|   IBIS model for TI xxx DSP
[IBIS Ver]   5.1
[Disclaimer]   Please be aware that in the absence of a written agreement
|   Texas Instruments(TI) assumes no liability for:
|   (1) The accuracy of the IBIS models provided to your company,
|   however, the IBIS model is compliant to industry standard
|   IQ Level 2a.  Refer to IBIS Quality Section below for
|   for full details.
|   (2) The proper functioning of these Models in your design
|   or for any resulting applications
|   (3) Infringement of patents, copyrights or intellectual
|   property rights resulting from your use of these
|   models.
|   TI provides IBIS Models as a service to our customers and
|   therefore reserves the right to limit distribution of the
|   Models.  The information is subject to change without notice.
[File Name]  am64_ani.ibs
[File Rev]   0.1
|   - Initial version
[Date]   3 Nov 2025
[Source]   Texas Instruments Incorporated
[Copyright]   Property of Texas Instruments Incorporated.
|   Unauthorized reproduction and/or distribution is strictly.
|   prohibited.
|   This product is protected under copyright law and trade
|   secret law as an unpublished work.
|   Created 2012,(C) Copyright 1999-2012,
|   Texas Instruments Incorporated., All Rights Reserved.
|   These commodities are under the U.S. Government
|   distribution license control. As such,they are not to be
|   re-exported without the prior approval of the U.S.
|   Department of Commerce.
[Notes]
   This file does not include AMI models for SerDes based links.
   For SerDes simulations use Texas Instruments IBIS AMI models
   Some IV curves contain Non monotonic data points.
|   Revision History
|   GERNERAL COMMENT: All IBIS Quality Notes below reflect latest release
|   and version of IBIS File
|   File passes ibischk5.1 and ibischk6 with 0 errors and 66 warnings
|   Component AM64
[Component] AM64
[Manufacturer] Texas Instruments
[Package]
|Variable   Typ   Min   Max
R_pkg   0.36429   0.078021   0.69181
L_pkg   2.771e-9   9.357e-10   5.062e-9
C_pkg   1.024e-12   5.807e-13   1.505e-12
[Package Model]   am64_ani_pkg
[Pin]  Signal_name   model_name
G20	ADC0_AIN0		NC
F20	ADC0_AIN1		NC
E21	ADC0_AIN2		NC
D20	ADC0_AIN3		NC
G21	ADC0_AIN4		NC
F21	ADC0_AIN5		NC
F19	ADC0_AIN6		NC
E20	ADC0_AIN7		NC
J16	ADC0_REFN		NC
J15	ADC0_REFP		NC
G13	ATEST0			NC
D2	DDR0_A0			DDR_SE
C5	DDR0_A1			DDR_SE
K3	DDR0_A10		DDR_SE
J1	DDR0_A11		DDR_SE
M5	DDR0_A12		DDR_SE
K4	DDR0_A13		DDR_SE
E2	DDR0_A2			DDR_SE
D4	DDR0_A3			DDR_SE
D3	DDR0_A4			DDR_SE
F2	DDR0_A5			DDR_SE
J2	DDR0_A6			DDR_SE
L5	DDR0_A7			DDR_SE
J3	DDR0_A8			DDR_SE
J4	DDR0_A9			DDR_SE
H2	DDR0_ACT_N		DDR_SE
H1	DDR0_ALERT_N   DDR_SE
K2	DDR0_ATB0		DDR_SE
K1	DDR0_ATB1		DDR_SE
G4	DDR0_BA0		DDR_SE
G5	DDR0_BA1		DDR_SE
G2	DDR0_BG0		DDR_SE
H3	DDR0_BG1		DDR_SE
H5	DDR0_CAL0		DDR_SE
J5	DDR0_CAS_N		DDR_SE
F1	DDR0_CK0		DDR_DIFF
E1	DDR0_CK0_N		DDR_DIFF
F4	DDR0_CKE0		DDR_SE
F3	DDR0_CKE1		DDR_SE
E3	DDR0_CS0_N		DDR_SE
E4	DDR0_CS1_N		DDR_SE
B2	DDR0_DM0		DDR_SE
M2	DDR0_DM1   DDR_SE
A3	DDR0_DQ0   DDR_SE
A2	DDR0_DQ1   DDR_SE
L2	DDR0_DQ10   DDR_SE
M3	DDR0_DQ11   DDR_SE
N4	DDR0_DQ12   DDR_SE
N3	DDR0_DQ13   DDR_SE
M4	DDR0_DQ14   DDR_SE
N2	DDR0_DQ15   DDR_SE
B5	DDR0_DQ2   DDR_SE
A4	DDR0_DQ3   DDR_SE
B3	DDR0_DQ4   DDR_SE
C4	DDR0_DQ5   DDR_SE
C2	DDR0_DQ6   DDR_SE
B4	DDR0_DQ7   DDR_SE
N5	DDR0_DQ8   DDR_SE
L4	DDR0_DQ9   DDR_SE
C1	DDR0_DQS0   DDR_DIFF
B1	DDR0_DQS0_N   DDR_DIFF
N1	DDR0_DQS1   DDR_DIFF
M1	DDR0_DQS1_N   DDR_DIFF
E5	DDR0_ODT0   DDR_SE
F5	DDR0_ODT1   DDR_SE
K5	DDR0_PAR   DDR_SE
F6	DDR0_RAS_N   DDR_SE
D5	DDR0_RESET0_N   DDR_SE
H4	DDR0_WE_N   DDR_SE
D18	ECAP0_IN_APWM_OUT	LVCMOS_V
D10	EMU0   LVCMOS_V
E10	EMU1   LVCMOS_V
A19	EXT_REFCLK1   LVCMOS_V
C19	EXTINTN   IIC_V
T20	GPMC0_AD0   LVCMOS_H
U21	GPMC0_AD1   LVCMOS_H
R16	GPMC0_AD10   LVCMOS_H
W20	GPMC0_AD11   LVCMOS_H
W21	GPMC0_AD12   LVCMOS_H
V18	GPMC0_AD13   LVCMOS_H
Y21	GPMC0_AD14   LVCMOS_H
Y20	GPMC0_AD15   LVCMOS_H
T18	GPMC0_AD2   LVCMOS_H
U20	GPMC0_AD3   LVCMOS_H
U18	GPMC0_AD4   LVCMOS_H
U19	GPMC0_AD5   LVCMOS_H
V20	GPMC0_AD6   LVCMOS_H
V21	GPMC0_AD7   LVCMOS_H
V19	GPMC0_AD8   LVCMOS_H
T17	GPMC0_AD9   LVCMOS_H
P16	GPMC0_ADVN_ALE   LVCMOS_H
P17	GPMC0_BE0N_CLE   LVCMOS_H
T19	GPMC0_BE1N   LVCMOS_H
R17	GPMC0_CLK   LVCMOS_H
R19	GPMC0_CSN0   LVCMOS_H
R20	GPMC0_CSN1   LVCMOS_H
P19	GPMC0_CSN2   LVCMOS_H
R21	GPMC0_CSN3   LVCMOS_H
N17	GPMC0_DIR   LVCMOS_H
R18	GPMC0_OEN_REN   LVCMOS_H
W19	GPMC0_WAIT0   LVCMOS_H
Y18	GPMC0_WAIT1   LVCMOS_H
T21	GPMC0_WEN   LVCMOS_H
N16	GPMC0_WPN   LVCMOS_H
A18	I2C0_SCL   IIC_V
B18	I2C0_SDA   IIC_V
C18	I2C1_SCL   LVCMOS_V
B19	I2C1_SDA   LVCMOS_V
H16	IFORCE   NC
B17	MCAN0_RX   LVCMOS_V
A17	MCAN0_TX   LVCMOS_V
D17	MCAN1_RX   LVCMOS_V
C17	MCAN1_TX   LVCMOS_V
E9	MCU_I2C0_SCL   IIC_V
A10	MCU_I2C0_SDA   IIC_V
A11	MCU_I2C1_SCL   LVCMOS_V
B10	MCU_I2C1_SDA   LVCMOS_V
C21	MCU_OSC0_XI   NC
B20	MCU_OSC0_XO   NC
B21	MCU_PORZ   RESET_H
B13	MCU_RESETSTATZ   LVCMOS_V
B12	MCU_RESETZ   LVCMOS_V
A20	MCU_SAFETY_ERRORN	LVCMOS_V
E6	MCU_SPI0_CLK   LVCMOS_V
D6	MCU_SPI0_CS0   LVCMOS_V
C6	MCU_SPI0_CS1   LVCMOS_V
E7	MCU_SPI0_D0   LVCMOS_V
B6	MCU_SPI0_D1   LVCMOS_V
D7	MCU_SPI1_CLK   LVCMOS_V
A7	MCU_SPI1_CS0   LVCMOS_V
B7	MCU_SPI1_CS1   LVCMOS_V
C7	MCU_SPI1_D0   LVCMOS_V
C8	MCU_SPI1_D1   LVCMOS_V
D8	MCU_UART0_CTSN   LVCMOS_V
E8	MCU_UART0_RTSN   LVCMOS_V
A9	MCU_UART0_RXD   LVCMOS_V
A8	MCU_UART0_TXD   LVCMOS_V
B8	MCU_UART1_CTSN   LVCMOS_V
B9	MCU_UART1_RTSN   LVCMOS_V
C9	MCU_UART1_RXD   LVCMOS_V
D9	MCU_UART1_TXD   LVCMOS_V
F18	MMC0_CALPAD   EMMC
G18	MMC0_CLK   EMMC
J21	MMC0_CMD   EMMC
K20	MMC0_DAT0   EMMC
J20	MMC0_DAT1   EMMC
J18	MMC0_DAT2   EMMC
J17	MMC0_DAT3   EMMC
H17	MMC0_DAT4   EMMC
H19	MMC0_DAT5   EMMC
H18	MMC0_DAT6   EMMC
G17	MMC0_DAT7   EMMC
G19	MMC0_DS   EMMC
F17	MMC0_VCTRL_TP   EMMC
L20	MMC1_CLK   SDIO_H
J19	MMC1_CMD   SDIO_H
K21	MMC1_DAT0   SDIO_H
L21	MMC1_DAT1   SDIO_H
K19	MMC1_DAT2   SDIO_H
K18	MMC1_DAT3   SDIO_H
D19	MMC1_SDCD   LVCMOS_V
C20	MMC1_SDWP   LVCMOS_V
N20	OSPI0_CLK   LVCMOS_H
L19	OSPI0_CSN0   LVCMOS_H
L18	OSPI0_CSN1   LVCMOS_H
K17	OSPI0_CSN2   LVCMOS_H
L17	OSPI0_CSN3   LVCMOS_H
M19	OSPI0_D0   LVCMOS_H
M18	OSPI0_D1   LVCMOS_H
M20	OSPI0_D2   LVCMOS_H
M21	OSPI0_D3   LVCMOS_H
P21	OSPI0_D4   LVCMOS_H
P20	OSPI0_D5   LVCMOS_H
N18	OSPI0_D6   LVCMOS_H
M17	OSPI0_D7   LVCMOS_H
N19	OSPI0_DQS   LVCMOS_H
N21	OSPI0_LBCLKO   LVCMOS_H
E17	PORZ_OUT   LVCMOS_H
P3	PRG0_MDIO0_MDC   LVCMOS_H
P2	PRG0_MDIO0_MDIO   LVCMOS_H
Y1	PRG0_PRU0_GPO0   LVCMOS_H
R4	PRG0_PRU0_GPO1   LVCMOS_H
AA5	PRG0_PRU0_GPO10   LVCMOS_H
Y3	PRG0_PRU0_GPO11   LVCMOS_H
AA3	PRG0_PRU0_GPO12   LVCMOS_H
R6	PRG0_PRU0_GPO13   LVCMOS_H
V4	PRG0_PRU0_GPO14   LVCMOS_H
T5	PRG0_PRU0_GPO15   LVCMOS_H
U4	PRG0_PRU0_GPO16   LVCMOS_H
U1	PRG0_PRU0_GPO17   LVCMOS_H
V1	PRG0_PRU0_GPO18   LVCMOS_H
W1	PRG0_PRU0_GPO19   LVCMOS_H
U2	PRG0_PRU0_GPO2   LVCMOS_H
V2	PRG0_PRU0_GPO3   LVCMOS_H
AA2	PRG0_PRU0_GPO4   LVCMOS_H
R3	PRG0_PRU0_GPO5   LVCMOS_H
T3	PRG0_PRU0_GPO6   LVCMOS_H
T1	PRG0_PRU0_GPO7   LVCMOS_H
T2	PRG0_PRU0_GPO8   LVCMOS_H
W6	PRG0_PRU0_GPO9   LVCMOS_H
Y2	PRG0_PRU1_GPO0   LVCMOS_H
W2	PRG0_PRU1_GPO1   LVCMOS_H
V6	PRG0_PRU1_GPO10   LVCMOS_H
W4	PRG0_PRU1_GPO11   LVCMOS_H
Y4	PRG0_PRU1_GPO12   LVCMOS_H
T6	PRG0_PRU1_GPO13   LVCMOS_H
U6	PRG0_PRU1_GPO14   LVCMOS_H
U5	PRG0_PRU1_GPO15   LVCMOS_H
AA4	PRG0_PRU1_GPO16   LVCMOS_H
V5	PRG0_PRU1_GPO17   LVCMOS_H
P5	PRG0_PRU1_GPO18   LVCMOS_H
R2	PRG0_PRU1_GPO19   LVCMOS_H
V3	PRG0_PRU1_GPO2   LVCMOS_H
T4	PRG0_PRU1_GPO3   LVCMOS_H
W3	PRG0_PRU1_GPO4   LVCMOS_H
P4	PRG0_PRU1_GPO5   LVCMOS_H
R5	PRG0_PRU1_GPO6   LVCMOS_H
W5	PRG0_PRU1_GPO7   LVCMOS_H
R1	PRG0_PRU1_GPO8   LVCMOS_H
Y5	PRG0_PRU1_GPO9   LVCMOS_H
Y6	PRG1_MDIO0_MDC   LVCMOS_V
AA6	PRG1_MDIO0_MDIO   LVCMOS_V
Y7	PRG1_PRU0_GPO0   LVCMOS_V
U8	PRG1_PRU0_GPO1   LVCMOS_V
U14	PRG1_PRU0_GPO10   LVCMOS_V
AA8	PRG1_PRU0_GPO11   LVCMOS_V
U9	PRG1_PRU0_GPO12   LVCMOS_V
W9	PRG1_PRU0_GPO13   LVCMOS_V
AA9	PRG1_PRU0_GPO14   LVCMOS_V
Y9	PRG1_PRU0_GPO15   LVCMOS_V
V9	PRG1_PRU0_GPO16   LVCMOS_V
U7	PRG1_PRU0_GPO17   LVCMOS_V
V7	PRG1_PRU0_GPO18   LVCMOS_V
W7	PRG1_PRU0_GPO19   LVCMOS_V
W8	PRG1_PRU0_GPO2   LVCMOS_V
V8	PRG1_PRU0_GPO3   LVCMOS_V
Y8	PRG1_PRU0_GPO4   LVCMOS_V
V13	PRG1_PRU0_GPO5   LVCMOS_V
AA7	PRG1_PRU0_GPO6   LVCMOS_V
U13	PRG1_PRU0_GPO7   LVCMOS_V
W13	PRG1_PRU0_GPO8   LVCMOS_V
U15	PRG1_PRU0_GPO9   LVCMOS_V
W11	PRG1_PRU1_GPO0   LVCMOS_V
V11	PRG1_PRU1_GPO1   LVCMOS_V
W14	PRG1_PRU1_GPO10   LVCMOS_V
AA10	PRG1_PRU1_GPO11   LVCMOS_V
V10	PRG1_PRU1_GPO12   LVCMOS_V
U10	PRG1_PRU1_GPO13   LVCMOS_V
AA11	PRG1_PRU1_GPO14   LVCMOS_V
Y11	PRG1_PRU1_GPO15   LVCMOS_V
Y10	PRG1_PRU1_GPO16   LVCMOS_V
AA14	PRG1_PRU1_GPO17   LVCMOS_V
Y13	PRG1_PRU1_GPO18   LVCMOS_V
V12	PRG1_PRU1_GPO19   LVCMOS_V
AA12	PRG1_PRU1_GPO2   LVCMOS_V
Y12	PRG1_PRU1_GPO3   LVCMOS_V
W12	PRG1_PRU1_GPO4   LVCMOS_V
AA13	PRG1_PRU1_GPO5   LVCMOS_V
U11	PRG1_PRU1_GPO6   LVCMOS_V
V15	PRG1_PRU1_GPO7   LVCMOS_V
U12	PRG1_PRU1_GPO8   LVCMOS_V
V14	PRG1_PRU1_GPO9   LVCMOS_V
E18	RESET_REQZ   LVCMOS_V
F16	RESETSTATZ   LVCMOS_V
W15	SERDES0_ATB_0   NC
V16	SERDES0_ATB_1   NC
W16	SERDES0_REFCLK0N	NC
W17	SERDES0_REFCLK0P	NC
T13	SERDES0_REXT   NC
Y15	SERDES0_RX0_N   NC
Y16	SERDES0_RX0_P   NC
AA16	SERDES0_TX0_N   NC
AA17	SERDES0_TX0_P   NC
D13	SPI0_CLK   LVCMOS_V
D12	SPI0_CS0   LVCMOS_V
C13	SPI0_CS1   LVCMOS_V
A13	SPI0_D0   LVCMOS_V
A14	SPI0_D1   LVCMOS_V
C14	SPI1_CLK   LVCMOS_V
B14	SPI1_CS0   LVCMOS_V
D14	SPI1_CS1   LVCMOS_V
B15	SPI1_D0   LVCMOS_V
A15	SPI1_D1   LVCMOS_V
B11	TCK   LVCMOS_V
C11	TDI   LVCMOS_V
A12	TDO   LVCMOS_V
F12	TEMP_DIODE_P   NC
C12	TMS   LVCMOS_V
D11	TRSTN   LVCMOS_V
B16	UART0_CTSN   LVCMOS_V
A16	UART0_RTSN   LVCMOS_V
D15	UART0_RXD   LVCMOS_V
C16	UART0_TXD   LVCMOS_V
D16	UART1_CTSN   LVCMOS_V
E16	UART1_RTSN   LVCMOS_V
E15	UART1_RXD   LVCMOS_V
E14	UART1_TXD   LVCMOS_V
AA20	USB0_DM   NC
AA19	USB0_DP   NC
E19	USB0_DRVVBUS   LVCMOS_V
U16	USB0_ID   NC
U17	USB0_RCALIB   NC
T14	USB0_VBUS   NC
D21	VSENSE   NC
Y19   VSS   GND
Y17   VSS   GND
Y14   VSS   GND
W18   VSS   GND
W10   VSS   GND
V17   VSS   GND
U3   VSS   GND
T8   VSS   GND
T16   VSS   GND
T15   VSS   GND
T11   VSS   GND
T10   VSS   GND
R9   VSS   GND
R7   VSS   GND
R12   VSS   GND
P8   VSS   GND
P6   VSS   GND
P18   VSS   GND
P10   VSS   GND
P1   VSS   GND
N9   VSS   GND
N7   VSS   GND
N15   VSS   GND
N13   VSS   GND
N11   VSS   GND
M8   VSS   GND
M6   VSS   GND
M12   VSS   GND
M10   VSS   GND
L9   VSS   GND
L7   VSS   GND
L3   VSS   GND
L16   VSS   GND
L1   VSS   GND
K8   VSS   GND
K6   VSS   GND
J9   VSS   GND
J7   VSS   GND
J14   VSS   GND
H8   VSS   GND
H6   VSS   GND
H21   VSS   GND
H20   VSS   GND
H11   VSS   GND
G9   VSS   GND
G7   VSS   GND
G3   VSS   GND
G16   VSS   GND
G1   VSS   GND
F8   VSS   GND
F15   VSS   GND
F10   VSS   GND
E13   VSS   GND
E11   VSS   GND
D1   VSS   GND
C3   VSS   GND
C15   VSS   GND
C10   VSS   GND
AA21   VSS   GND
AA18   VSS   GND
AA15   VSS   GND
AA1   VSS   GND
A6   VSS   GND
A5   VSS   GND
A21   VSS   GND
A1   VSS   GND
H12   CAP_VDDS0   POWER
T7   CAP_VDDS1   POWER
R11   CAP_VDDS2   POWER
N14   CAP_VDDS3   POWER
M16   CAP_VDDS4   POWER
L13   CAP_VDDS5   POWER
K15   CAP_VDDSHV_MMC1   POWER
H10   CAP_VDDS_MCU   POWER
P13   VDDA_0P85_SERDES0   POWER
P12   VDDA_0P85_SERDES0   POWER
P11   VDDA_0P85_SERDES0_C   POWER
T12   VDDA_0P85_USB0   POWER
R14   VDDA_1P8_SERDES0   POWER
R15   VDDA_1P8_USB0   POWER
H15   VDDA_3P3_SDIO   POWER
R13   VDDA_3P3_USB0   POWER
J13   VDDA_ADC   POWER
K12   VDDA_MCU   POWER
N12   VDDA_PLL0   POWER
H9   VDDA_PLL1   POWER
J11   VDDA_PLL2   POWER
G11   VDDA_TEMP0   POWER
L11   VDDA_TEMP1   POWER
M13   VDDR_CORE   POWER
L10   VDDR_CORE   POWER
G14   VDDSHV0   POWER
G12   VDDSHV0   POWER
F11   VDDSHV0   POWER
P7   VDDSHV1   POWER
N6   VDDSHV1   POWER
M7   VDDSHV1   POWER
T9   VDDSHV2   POWER
R8   VDDSHV2   POWER
R10   VDDSHV2   POWER
P15   VDDSHV3   POWER
P14   VDDSHV3   POWER
M15   VDDSHV4   POWER
M14   VDDSHV4   POWER
L15   VDDSHV5   POWER
L14   VDDSHV5   POWER
G8   VDDSHV_MCU   POWER
G10   VDDSHV_MCU   POWER
F9   VDDSHV_MCU   POWER
L6   VDDS_DDR   POWER
K7   VDDS_DDR   POWER
J6   VDDS_DDR   POWER
H7   VDDS_DDR   POWER
G6   VDDS_DDR   POWER
F7   VDDS_DDR   POWER
J8   VDDS_DDR_C   POWER
K14   VDDS_MMC0   POWER
H13   VDDS_OSC   POWER
P9   VDD_CORE   POWER
N8   VDD_CORE   POWER
N10   VDD_CORE   POWER
M9   VDD_CORE   POWER
M11   VDD_CORE   POWER
L8   VDD_CORE   POWER
L12   VDD_CORE   POWER
K9   VDD_CORE   POWER
K11   VDD_CORE   POWER
J12   VDD_CORE   POWER
J10   VDD_CORE   POWER
H14   VDD_DLL_MMC0   POWER
K13   VDD_MMC0   POWER
K16   VMON_1P8_MCU   POWER
E12   VMON_1P8_SOC   POWER
F13   VMON_3P3_MCU   POWER
F14   VMON_3P3_SOC   POWER
K10   VMON_VSYS   POWER
G15   VPP   POWER
|********************  DIFF PIN  *******************************
[Diff_pin]   inv_pin vdiff tdelay_typ   tdelay_min  tdelay_max
C1	B1	NA NA NA NA	||	DDR0_DQS0	&	DDR0_DQS0_N
N1	M1	NA NA NA NA	||	DDR0_DQS1	&	DDR0_DQS1_N
F1	E1	NA NA NA NA	||	DDR0_CK0	&	DDR0_CK0_N
|---------------- DDR -------------------
[Model Selector] DDR_SE
lpddr4_ocd_240p_240n  driver with 240 ohms pullup and 240 ohms pulldown strength
lpddr4_ocd_120p_120n  driver with 120 ohms pullup and 120 ohms pulldown strength
lpddr4_ocd_80p_80n  driver with 80 ohms pullup and 80 ohms pulldown strength
lpddr4_ocd_60p_60n  driver with 60 ohms pullup and 60 ohms pulldown strength
lpddr4_ocd_48p_48n  driver with 48 ohms pullup and 48 ohms pulldown strength
lpddr4_ocd_40p_40n  driver with 40 ohms pullup and 40 ohms pulldown strength
lpddr4_ocd_120pd_60p_40n  driver with 60/40 ohms pullup/pulldown 120 ohms aopd strength
lpddr4_ocd_120pd_48p_40n  driver with 48/40 ohms pullup/pulldown 120 ohms aopd strength
lp4x_ocd_34p_34n  driver with 34 ohms pullup and 34 ohms pulldown strength
lp4x_ocd_40p_40n  driver with 40 ohms pullup and 40 ohms pulldown strength
lp4x_ocd_48p_48n  driver with 48 ohms pullup and 48 ohms pulldown strength
lp4x_ocd_60p_60n  driver with 60 ohms pullup and 60 ohms pulldown strength
lp4x_ocd_80p_80n  driver with 80 ohms pullup and 80 ohms pulldown strength
lp4x_ocd_120p_120n  driver with 120 ohms pullup and 120 ohms pulldown strength
lp4x_ocd_240p_240n  driver with 240 ohms pullup and 240 ohms pulldown strength
lp4x_0p6_ocd_80p_80n  driver with 80 ohms pullup and 80 ohms pulldown strength
lp4x_0p6_ocd_40p_40n  driver with 40 ohms pullup and 40 ohms pulldown strength
lpddr4_odt_240  240 ohm termination
lpddr4_odt_120  120 ohm termination
lpddr4_odt_80  80 ohm termination
lpddr4_odt_60  60 ohm termination
lpddr4_odt_48  48 ohm termination
lpddr4_odt_40  40 ohm termination
lpddr4_odt_off  open ohm termination
lp4x_odt_40  40 ohm termination
lp4x_odt_48  48 ohm termination
lp4x_odt_60  60 ohm termination
lp4x_odt_80  80 ohm termination
lp4x_odt_120  120 ohm termination
lp4x_odt_240  240 ohm termination
lp4x_odt_off  open
ddr4_ocd_34p_34n  driver with 34 ohms pullup and 34 ohms pulldown strength, max slew rate
ddr4_ocd_40p_40n  driver with 40 ohms pullup and 40 ohms pulldown strength, max slew rate
ddr4_ocd_48p_48n  driver with 48 ohms pullup and 48 ohms pulldown strength, max slew rate
ddr4_ocd_60p_60n  driver with 60 ohms pullup and 60 ohms pulldown strength, max slew rate
ddr4_ocd_80p_80n  driver with 80 ohms pullup and 80 ohms pulldown strength, max slew rate
ddr4_odt_34  34 ohm termination
ddr4_odt_40  40 ohm termination
ddr4_odt_48  48 ohm termination
ddr4_odt_60  60 ohm termination
ddr4_odt_80  80 ohm termination
ddr4_odt_120  120 ohm termination
ddr4_odt_240  240 ohm termination
ddr4_odt_off  No termination
[Model Selector] DDR_DIFF
lpddr4_ocd_240p_240n_diff  driver with 240 ohms pullup and 240 ohms pulldown strength
lpddr4_ocd_120p_120n_diff  driver with 120 ohms pullup and 120 ohms pulldown strength
lpddr4_ocd_80p_80n_diff  driver with 80 ohms pullup and 80 ohms pulldown strength
lpddr4_ocd_60p_60n_diff  driver with 60 ohms pullup and 60 ohms pulldown strength
lpddr4_ocd_48p_48n_diff  driver with 48 ohms pullup and 48 ohms pulldown strength
lpddr4_ocd_40p_40n_diff  driver with 40 ohms pullup and 40 ohms pulldown strength
lpddr4_ocd_120pd_60p_40n_diff  driver with 60/40 ohms pullup/pulldown 120 ohms aopd strength
lpddr4_ocd_120pd_48p_40n_diff  driver with 48/40 ohms pullup/pulldown 120 ohms aopd strength
lp4x_ocd_34p_34n_diff  driver with 34 ohms pullup and 34 ohms pulldown strength
lp4x_ocd_40p_40n_diff  driver with 40 ohms pullup and 40 ohms pulldown strength
lp4x_ocd_48p_48n_diff  driver with 48 ohms pullup and 48 ohms pulldown strength
lp4x_ocd_60p_60n_diff  driver with 60 ohms pullup and 60 ohms pulldown strength
lp4x_ocd_80p_80n_diff  driver with 80 ohms pullup and 80 ohms pulldown strength
lp4x_ocd_120p_120n_diff  driver with 120 ohms pullup and 120 ohms pulldown strength
lp4x_ocd_240p_240n_diff  driver with 240 ohms pullup and 240 ohms pulldown strength
lp4x_0p6_ocd_80p_80n_diff  driver with 80 ohms pullup and 80 ohms pulldown strength
lp4x_0p6_ocd_40p_40n_diff  driver with 40 ohms pullup and 40 ohms pulldown strength
lpddr4_odt_240_diff  240 ohm termination
lpddr4_odt_120_diff  120 ohm termination
lpddr4_odt_80_diff  80 ohm termination
lpddr4_odt_60_diff  60 ohm termination
lpddr4_odt_48_diff  48 ohm termination
lpddr4_odt_40_diff  40 ohm termination
lpddr4_odt_off_diff  open ohm termination
lp4x_odt_40_diff  40 ohm termination
lp4x_odt_48_diff  48 ohm termination
lp4x_odt_60_diff  60 ohm termination
lp4x_odt_80_diff  80 ohm termination
lp4x_odt_120_diff  120 ohm termination
lp4x_odt_240_diff  240 ohm termination
lp4x_odt_off_diff  open
ddr4_ocd_34p_34n_diff  driver with 34 ohms pullup and 34 ohms pulldown strength, max slew rate
ddr4_ocd_40p_40n_diff  driver with 40 ohms pullup and 40 ohms pulldown strength, max slew rate
ddr4_ocd_48p_48n_diff  driver with 48 ohms pullup and 48 ohms pulldown strength, max slew rate
ddr4_ocd_60p_60n_diff  driver with 60 ohms pullup and 60 ohms pulldown strength, max slew rate
ddr4_ocd_80p_80n_diff  driver with 80 ohms pullup and 80 ohms pulldown strength, max slew rate
ddr4_odt_34_diff  34 ohm termination
ddr4_odt_40_diff  40 ohm termination
ddr4_odt_48_diff  48 ohm termination
ddr4_odt_60_diff  60 ohm termination
ddr4_odt_80_diff  80 ohm termination
ddr4_odt_120_diff  120 ohm termination
ddr4_odt_240_diff  240 ohm termination
ddr4_odt_off_diff  No termination
|****************** SDIO
[Model Selector] SDIO_H
sdio1_r40_1p8_h PRWDWUWSWEWCDGSDIO_H@_R40_1p8_comment
sdio1_r40_3p3_h PRWDWUWSWEWCDGSDIO_H@_R40_3p3_comment
|********** LVCMOS
[Model Selector] LVCMOS_H
lvcmos1_nom_1p8_h PRWDWUWSWEWCDGLVCMOS_H@_Nom_1p8_comment
lvcmos1_nom_3p3_h PRWDWUWSWEWCDGLVCMOS_H@_Nom_3p3_comment
lvcmos1_fast_1p8_h PRWDWUWSWEWCDGLVCMOS_H@_Fast_1p8_comment
lvcmos1_fast_3p3_h PRWDWUWSWEWCDGLVCMOS_H@_Fast_3p3_comment
[Model Selector] LVCMOS_V
lvcmos0_nom_1p8_v PRWDWUWSWEWCDGLVCMOS_V@_Nom_1p8_comment
lvcmos0_nom_3p3_v PRWDWUWSWEWCDGLVCMOS_V@_Nom_3p3_comment
lvcmos0_fast_1p8_v PRWDWUWSWEWCDGLVCMOS_V@_Fast_1p8_comment
lvcmos0_fast_3p3_v PRWDWUWSWEWCDGLVCMOS_V@_Fast_3p3_comment
[Model Selector] IIC_V
IIC18_1_0_V PRBOPDDGZIIC_V@HSMODE_HSMCSE=0_0_comment 1.8V
IIC18_1_1_V PRBOPDDGZIIC_V@HSMODE_HSMCSE=0_1_comment 1.8V
IIC18_1_2_V PRBOPDDGZIIC_V@HSMODE_HSMCSE=1_0_comment 1.8V
IIC18_1_3_V PRBOPDDGZIIC_V@HSMODE_HSMCSE=1_1_comment 1.8V
IIC33_1_0_V PRBOPDDGZIIC_V@HSMODE_HSMCSE=0_0_comment
|***************** RESET ************************************************
[Model Selector] RESET_H
reset18_0_0 PDIDGZRESET_H
|   EMMC
[MODEL SELECTOR] EMMC
emmc51_io_tx50ohm   50ohm DRIVE
|   Package Model
[Define Package Model]   am64_ani_pkg
[Manufacturer]   name 1
[OEM]   name 2
[Description]   347-pin Package
|[Number of Sections]   1
[Number of Pins]   347
[Pin Numbers]
|[Pin Name]  Net Number   Net Name   Net's All Pins
H12   | 1   CAP_VDDS0   H12
T7   | 2   CAP_VDDS1   T7
R11   | 3   CAP_VDDS2   R11
N14   | 4   CAP_VDDS3   N14
M16   | 5   CAP_VDDS4   M16
L13   | 6   CAP_VDDS5   L13
K15   | 7   CAP_VDDSHV_MMC1   K15
H10   | 8   CAP_VDDS_MCU   H10
P12   | 9   VDDA_0P85_SERDES0   P12
   |P13
P11   | 10   VDDA_0P85_SERDES0_C   P11
T12   | 11   VDDA_0P85_USB0   T12
R14   | 12   VDDA_1P8_SERDES0   R14
R15   | 13   VDDA_1P8_USB0   R15
H15   | 14   VDDA_3P3_SDIO   H15
R13   | 15   VDDA_3P3_USB0   R13
J13   | 16   VDDA_ADC   J13
K12   | 17   VDDA_MCU   K12
N12   | 18   VDDA_PLL0   N12
H9   | 19   VDDA_PLL1   H9
J11   | 20   VDDA_PLL2   J11
G11   | 21   VDDA_TEMP0   G11
L11   | 22   VDDA_TEMP1   L11
L10   | 23   VDDR_CORE   L10
   |M13
F11   | 24   VDDSHV0   F11
   |G12
   |G14
M7   | 25   VDDSHV1   M7
   |N6
   |P7
R8   | 26   VDDSHV2   R8
   |R10
   |T9
P14   | 27   VDDSHV3   P14
   |P15
M14   | 28   VDDSHV4   M14
   |M15
L14   | 29   VDDSHV5   L14
   |L15
F9   | 30   VDDSHV_MCU   F9
   |G8
   |G10
F7   | 31   VDDS_DDR   F7
   |G6
   |H7
   |J6
   |K7
   |L6
J8   | 32   VDDS_DDR_C   J8
K14   | 33   VDDS_MMC0   K14
H13   | 34   VDDS_OSC   H13
J10   | 35   VDD_CORE   J10
   |J12
   |K9
   |K11
   |L8
   |L12
   |M9
   |M11
   |N8
   |N10
   |P9
H14   | 36   VDD_DLL_MMC0   H14
K13   | 37   VDD_MMC0   K13
G15   | 38   VPP   G15
G20   | 39   ADC0_AIN0   G20
F20   | 40   ADC0_AIN1   F20
E21   | 41   ADC0_AIN2   E21
D20   | 42   ADC0_AIN3   D20
G21   | 43   ADC0_AIN4   G21
F21   | 44   ADC0_AIN5   F21
F19   | 45   ADC0_AIN6   F19
E20   | 46   ADC0_AIN7   E20
J16   | 47   ADC0_REFN   J16
J15   | 48   ADC0_REFP   J15
G13   | 49   ATEST0   G13
D2   | 50   DDR0_A0   D2
C5   | 51   DDR0_A1   C5
E2   | 52   DDR0_A2   E2
D4   | 53   DDR0_A3   D4
D3   | 54   DDR0_A4   D3
F2   | 55   DDR0_A5   F2
J2   | 56   DDR0_A6   J2
L5   | 57   DDR0_A7   L5
J3   | 58   DDR0_A8   J3
J4   | 59   DDR0_A9   J4
K3   | 60   DDR0_A10   K3
J1   | 61   DDR0_A11   J1
M5   | 62   DDR0_A12   M5
K4   | 63   DDR0_A13   K4
H2   | 64   DDR0_ACT_N   H2
H1   | 65   DDR0_ALERT_N   H1
K2   | 66   DDR0_ATB0   K2
K1   | 67   DDR0_ATB1   K1
G4   | 68   DDR0_BA0   G4
G5   | 69   DDR0_BA1   G5
G2   | 70   DDR0_BG0   G2
H3   | 71   DDR0_BG1   H3
H5   | 72   DDR0_CAL0   H5
J5   | 73   DDR0_CAS_N   J5
F1   | 74   DDR0_CK0   F1
E1   | 75   DDR0_CK0_N   E1
F4   | 76   DDR0_CKE0   F4
F3   | 77   DDR0_CKE1   F3
E3   | 78   DDR0_CS0_N   E3
E4   | 79   DDR0_CS1_N   E4
B2   | 80   DDR0_DM0   B2
M2   | 81   DDR0_DM1   M2
A3   | 82   DDR0_DQ0   A3
A2   | 83   DDR0_DQ1   A2
B5   | 84   DDR0_DQ2   B5
A4   | 85   DDR0_DQ3   A4
B3   | 86   DDR0_DQ4   B3
C4   | 87   DDR0_DQ5   C4
C2   | 88   DDR0_DQ6   C2
B4   | 89   DDR0_DQ7   B4
N5   | 90   DDR0_DQ8   N5
L4   | 91   DDR0_DQ9   L4
L2   | 92   DDR0_DQ10   L2
M3   | 93   DDR0_DQ11   M3
N4   | 94   DDR0_DQ12   N4
N3   | 95   DDR0_DQ13   N3
M4   | 96   DDR0_DQ14   M4
N2   | 97   DDR0_DQ15   N2
C1   | 98   DDR0_DQS0   C1
B1   | 99   DDR0_DQS0_N   B1
N1   | 100   DDR0_DQS1   N1
M1   | 101   DDR0_DQS1_N   M1
E5   | 102   DDR0_ODT0   E5
F5   | 103   DDR0_ODT1   F5
K5   | 104   DDR0_PAR   K5
F6   | 105   DDR0_RAS_N   F6
D5   | 106   DDR0_RESET0_N   D5
H4   | 107   DDR0_WE_N   H4
D18   | 108   ECAP0_IN_APWM_OUT   D18
D10   | 109   EMU0   D10
E10   | 110   EMU1   E10
C19   | 111   EXTINTN   C19
A19   | 112   EXT_REFCLK1   A19
T20   | 113   GPMC0_AD0   T20
U21   | 114   GPMC0_AD1   U21
T18   | 115   GPMC0_AD2   T18
U20   | 116   GPMC0_AD3   U20
U18   | 117   GPMC0_AD4   U18
U19   | 118   GPMC0_AD5   U19
V20   | 119   GPMC0_AD6   V20
V21   | 120   GPMC0_AD7   V21
V19   | 121   GPMC0_AD8   V19
T17   | 122   GPMC0_AD9   T17
R16   | 123   GPMC0_AD10   R16
W20   | 124   GPMC0_AD11   W20
W21   | 125   GPMC0_AD12   W21
V18   | 126   GPMC0_AD13   V18
Y21   | 127   GPMC0_AD14   Y21
Y20   | 128   GPMC0_AD15   Y20
P16   | 129   GPMC0_ADVN_ALE   P16
P17   | 130   GPMC0_BE0N_CLE   P17
T19   | 131   GPMC0_BE1N   T19
R17   | 132   GPMC0_CLK   R17
R19   | 133   GPMC0_CSN0   R19
R20   | 134   GPMC0_CSN1   R20
P19   | 135   GPMC0_CSN2   P19
R21   | 136   GPMC0_CSN3   R21
N17   | 137   GPMC0_DIR   N17
R18   | 138   GPMC0_OEN_REN   R18
W19   | 139   GPMC0_WAIT0   W19
Y18   | 140   GPMC0_WAIT1   Y18
T21   | 141   GPMC0_WEN   T21
N16   | 142   GPMC0_WPN   N16
A18   | 143   I2C0_SCL   A18
B18   | 144   I2C0_SDA   B18
C18   | 145   I2C1_SCL   C18
B19   | 146   I2C1_SDA   B19
H16   | 147   IFORCE   H16
B17   | 148   MCAN0_RX   B17
A17   | 149   MCAN0_TX   A17
D17   | 150   MCAN1_RX   D17
C17   | 151   MCAN1_TX   C17
E9   | 152   MCU_I2C0_SCL   E9
A10   | 153   MCU_I2C0_SDA   A10
A11   | 154   MCU_I2C1_SCL   A11
B10   | 155   MCU_I2C1_SDA   B10
C21   | 156   MCU_OSC0_XI   C21
B20   | 157   MCU_OSC0_XO   B20
B21   | 158   MCU_PORZ   B21
B13   | 159   MCU_RESETSTATZ   B13
B12   | 160   MCU_RESETZ   B12
A20   | 161   MCU_SAFETY_ERRORN   A20
E6   | 162   MCU_SPI0_CLK   E6
D6   | 163   MCU_SPI0_CS0   D6
C6   | 164   MCU_SPI0_CS1   C6
E7   | 165   MCU_SPI0_D0   E7
B6   | 166   MCU_SPI0_D1   B6
D7   | 167   MCU_SPI1_CLK   D7
A7   | 168   MCU_SPI1_CS0   A7
B7   | 169   MCU_SPI1_CS1   B7
C7   | 170   MCU_SPI1_D0   C7
C8   | 171   MCU_SPI1_D1   C8
D8   | 172   MCU_UART0_CTSN   D8
E8   | 173   MCU_UART0_RTSN   E8
A9   | 174   MCU_UART0_RXD   A9
A8   | 175   MCU_UART0_TXD   A8
B8   | 176   MCU_UART1_CTSN   B8
B9   | 177   MCU_UART1_RTSN   B9
C9   | 178   MCU_UART1_RXD   C9
D9   | 179   MCU_UART1_TXD   D9
F18   | 180   MMC0_CALPAD   F18
G18   | 181   MMC0_CLK   G18
J21   | 182   MMC0_CMD   J21
K20   | 183   MMC0_DAT0   K20
J20   | 184   MMC0_DAT1   J20
J18   | 185   MMC0_DAT2   J18
J17   | 186   MMC0_DAT3   J17
H17   | 187   MMC0_DAT4   H17
H19   | 188   MMC0_DAT5   H19
H18   | 189   MMC0_DAT6   H18
G17   | 190   MMC0_DAT7   G17
G19   | 191   MMC0_DS   G19
F17   | 192   MMC0_VCTRL_TP   F17
L20   | 193   MMC1_CLK   L20
J19   | 194   MMC1_CMD   J19
K21   | 195   MMC1_DAT0   K21
L21   | 196   MMC1_DAT1   L21
K19   | 197   MMC1_DAT2   K19
K18   | 198   MMC1_DAT3   K18
D19   | 199   MMC1_SDCD   D19
C20   | 200   MMC1_SDWP   C20
N20   | 201   OSPI0_CLK   N20
L19   | 202   OSPI0_CSN0   L19
L18   | 203   OSPI0_CSN1   L18
K17   | 204   OSPI0_CSN2   K17
L17   | 205   OSPI0_CSN3   L17
M19   | 206   OSPI0_D0   M19
M18   | 207   OSPI0_D1   M18
M20   | 208   OSPI0_D2   M20
M21   | 209   OSPI0_D3   M21
P21   | 210   OSPI0_D4   P21
P20   | 211   OSPI0_D5   P20
N18   | 212   OSPI0_D6   N18
M17   | 213   OSPI0_D7   M17
N19   | 214   OSPI0_DQS   N19
N21   | 215   OSPI0_LBCLKO   N21
E17   | 216   PORZ_OUT   E17
P3   | 217   PRG0_MDIO0_MDC   P3
P2   | 218   PRG0_MDIO0_MDIO   P2
Y1   | 219   PRG0_PRU0_GPO0   Y1
R4   | 220   PRG0_PRU0_GPO1   R4
U2   | 221   PRG0_PRU0_GPO2   U2
V2   | 222   PRG0_PRU0_GPO3   V2
AA2   | 223   PRG0_PRU0_GPO4   AA2
R3   | 224   PRG0_PRU0_GPO5   R3
T3   | 225   PRG0_PRU0_GPO6   T3
T1   | 226   PRG0_PRU0_GPO7   T1
T2   | 227   PRG0_PRU0_GPO8   T2
W6   | 228   PRG0_PRU0_GPO9   W6
AA5   | 229   PRG0_PRU0_GPO10   AA5
Y3   | 230   PRG0_PRU0_GPO11   Y3
AA3   | 231   PRG0_PRU0_GPO12   AA3
R6   | 232   PRG0_PRU0_GPO13   R6
V4   | 233   PRG0_PRU0_GPO14   V4
T5   | 234   PRG0_PRU0_GPO15   T5
U4   | 235   PRG0_PRU0_GPO16   U4
U1   | 236   PRG0_PRU0_GPO17   U1
V1   | 237   PRG0_PRU0_GPO18   V1
W1   | 238   PRG0_PRU0_GPO19   W1
Y2   | 239   PRG0_PRU1_GPO0   Y2
W2   | 240   PRG0_PRU1_GPO1   W2
V3   | 241   PRG0_PRU1_GPO2   V3
T4   | 242   PRG0_PRU1_GPO3   T4
W3   | 243   PRG0_PRU1_GPO4   W3
P4   | 244   PRG0_PRU1_GPO5   P4
R5   | 245   PRG0_PRU1_GPO6   R5
W5   | 246   PRG0_PRU1_GPO7   W5
R1   | 247   PRG0_PRU1_GPO8   R1
Y5   | 248   PRG0_PRU1_GPO9   Y5
V6   | 249   PRG0_PRU1_GPO10   V6
W4   | 250   PRG0_PRU1_GPO11   W4
Y4   | 251   PRG0_PRU1_GPO12   Y4
T6   | 252   PRG0_PRU1_GPO13   T6
U6   | 253   PRG0_PRU1_GPO14   U6
U5   | 254   PRG0_PRU1_GPO15   U5
AA4   | 255   PRG0_PRU1_GPO16   AA4
V5   | 256   PRG0_PRU1_GPO17   V5
P5   | 257   PRG0_PRU1_GPO18   P5
R2   | 258   PRG0_PRU1_GPO19   R2
Y6   | 259   PRG1_MDIO0_MDC   Y6
AA6   | 260   PRG1_MDIO0_MDIO   AA6
Y7   | 261   PRG1_PRU0_GPO0   Y7
U8   | 262   PRG1_PRU0_GPO1   U8
W8   | 263   PRG1_PRU0_GPO2   W8
V8   | 264   PRG1_PRU0_GPO3   V8
Y8   | 265   PRG1_PRU0_GPO4   Y8
V13   | 266   PRG1_PRU0_GPO5   V13
AA7   | 267   PRG1_PRU0_GPO6   AA7
U13   | 268   PRG1_PRU0_GPO7   U13
W13   | 269   PRG1_PRU0_GPO8   W13
U15   | 270   PRG1_PRU0_GPO9   U15
U14   | 271   PRG1_PRU0_GPO10   U14
AA8   | 272   PRG1_PRU0_GPO11   AA8
U9   | 273   PRG1_PRU0_GPO12   U9
W9   | 274   PRG1_PRU0_GPO13   W9
AA9   | 275   PRG1_PRU0_GPO14   AA9
Y9   | 276   PRG1_PRU0_GPO15   Y9
V9   | 277   PRG1_PRU0_GPO16   V9
U7   | 278   PRG1_PRU0_GPO17   U7
V7   | 279   PRG1_PRU0_GPO18   V7
W7   | 280   PRG1_PRU0_GPO19   W7
W11   | 281   PRG1_PRU1_GPO0   W11
V11   | 282   PRG1_PRU1_GPO1   V11
AA12   | 283   PRG1_PRU1_GPO2   AA12
Y12   | 284   PRG1_PRU1_GPO3   Y12
W12   | 285   PRG1_PRU1_GPO4   W12
AA13   | 286   PRG1_PRU1_GPO5   AA13
U11   | 287   PRG1_PRU1_GPO6   U11
V15   | 288   PRG1_PRU1_GPO7   V15
U12   | 289   PRG1_PRU1_GPO8   U12
V14   | 290   PRG1_PRU1_GPO9   V14
W14   | 291   PRG1_PRU1_GPO10   W14
AA10   | 292   PRG1_PRU1_GPO11   AA10
V10   | 293   PRG1_PRU1_GPO12   V10
U10   | 294   PRG1_PRU1_GPO13   U10
AA11   | 295   PRG1_PRU1_GPO14   AA11
Y11   | 296   PRG1_PRU1_GPO15   Y11
Y10   | 297   PRG1_PRU1_GPO16   Y10
AA14   | 298   PRG1_PRU1_GPO17   AA14
Y13   | 299   PRG1_PRU1_GPO18   Y13
V12   | 300   PRG1_PRU1_GPO19   V12
F16   | 301   RESETSTATZ   F16
E18   | 302   RESET_REQZ   E18
W15   | 303   SERDES0_ATB_0   W15
V16   | 304   SERDES0_ATB_1   V16
W16   | 305   SERDES0_REFCLK0N   W16
W17   | 306   SERDES0_REFCLK0P   W17
T13   | 307   SERDES0_REXT   T13
Y15   | 308   SERDES0_RX0_N   Y15
Y16   | 309   SERDES0_RX0_P   Y16
AA16   | 310   SERDES0_TX0_N   AA16
AA17   | 311   SERDES0_TX0_P   AA17
D13   | 312   SPI0_CLK   D13
D12   | 313   SPI0_CS0   D12
C13   | 314   SPI0_CS1   C13
A13   | 315   SPI0_D0   A13
A14   | 316   SPI0_D1   A14
C14   | 317   SPI1_CLK   C14
B14   | 318   SPI1_CS0   B14
D14   | 319   SPI1_CS1   D14
B15   | 320   SPI1_D0   B15
A15   | 321   SPI1_D1   A15
B11   | 322   TCK   B11
C11   | 323   TDI   C11
A12   | 324   TDO   A12
F12   | 325   TEMP_DIODE_P   F12
C12   | 326   TMS   C12
D11   | 327   TRSTN   D11
B16   | 328   UART0_CTSN   B16
A16   | 329   UART0_RTSN   A16
D15   | 330   UART0_RXD   D15
C16   | 331   UART0_TXD   C16
D16   | 332   UART1_CTSN   D16
E16   | 333   UART1_RTSN   E16
E15   | 334   UART1_RXD   E15
E14   | 335   UART1_TXD   E14
AA20   | 336   USB0_DM   AA20
AA19   | 337   USB0_DP   AA19
E19   | 338   USB0_DRVVBUS   E19
U16   | 339   USB0_ID   U16
U17   | 340   USB0_RCALIB   U17
T14   | 341   USB0_VBUS   T14
K16   | 342   VMON_1P8_MCU   K16
E12   | 343   VMON_1P8_SOC   E12
F13   | 344   VMON_3P3_MCU   F13
F14   | 345   VMON_3P3_SOC   F14
K10   | 346   VMON_VSYS   K10
D21   | 347   VSENSE   D21
[Model Data]
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[End Model Data]
[End Package Model]
| Models and submodels in the file (119): lvcmos1_nom_1p8_h (I/O), lvcmos0_nom_1p8_v (I/O), lvcmos1_nom_3p3_h (I/O), lvcmos0_nom_3p3_v (I/O), lvcmos1_fast_1p8_h (I/O), lvcmos0_fast_1p8_v (I/O), lvcmos1_fast_3p3_h (I/O), lvcmos0_fast_3p3_v (I/O), sdio1_r33_1p8_h (I/O), sdio1_r33_3p3_h (I/O), sdio1_r40_1p8_h (I/O), sdio1_r40_3p3_h (I/O), sdio1_r50_1p8_h (I/O), sdio1_r50_3p3_h (I/O), sdio1_r66_1p8_h (I/O), sdio1_r66_3p3_h (I/O), lpddr4_odt_120 (Input), lpddr4_odt_120_diff (Input), lpddr4_ocd_120p_120n (I/O), lpddr4_ocd_240p_240n (I/O), lpddr4_odt_240 (Input), lpddr4_ocd_40p_40n (I/O), lpddr4_odt_40 (Input), lpddr4_ocd_48p_48n (I/O), lpddr4_odt_48 (Input), lpddr4_ocd_60p_60n (I/O), lpddr4_odt_60 (Input), lpddr4_ocd_80p_80n (I/O), lpddr4_odt_80 (Input), lpddr4_odt_off (Input), lpddr4_ocd_120pd_60p_40n (I/O), lpddr4_ocd_120p_120n_diff (I/O), lpddr4_ocd_240p_240n_diff (I/O), lpddr4_odt_240_diff (Input), lpddr4_ocd_40p_40n_diff (I/O), lpddr4_odt_40_diff (Input), lpddr4_ocd_48p_48n_diff (I/O), lpddr4_odt_48_diff (Input), lpddr4_ocd_60p_60n_diff (I/O), lpddr4_odt_60_diff (Input), lpddr4_ocd_80p_80n_diff (I/O), lpddr4_ocd_120pd_60p_40n_diff (I/O), lpddr4_odt_80_diff (Input), lpddr4_odt_off_diff (Input), lpddr4_ocd_120pd_48p_40n (I/O), lpddr4_ocd_120pd_48p_40n_diff (I/O), ddr4_ocd_34p_34n (I/O), ddr4_ocd_40p_40n (I/O), ddr4_ocd_48p_48n (I/O), ddr4_ocd_60p_60n (I/O), ddr4_ocd_80p_80n (I/O), ddr4_ocd_34p_34n_diff (I/O), ddr4_ocd_40p_40n_diff (I/O), ddr4_ocd_48p_48n_diff (I/O), ddr4_ocd_60p_60n_diff (I/O), ddr4_ocd_80p_80n_diff (I/O), ddr4_odt_34 (Input), ddr4_odt_40 (Input), ddr4_odt_48 (Input), ddr4_odt_60 (Input), ddr4_odt_80 (Input), ddr4_odt_120 (Input), ddr4_odt_240 (Input), ddr4_odt_off (Input), ddr4_odt_34_diff (Input), ddr4_odt_40_diff (Input), ddr4_odt_48_diff (Input), ddr4_odt_60_diff (Input), ddr4_odt_80_diff (Input), ddr4_odt_120_diff (Input), ddr4_odt_240_diff (Input), ddr4_odt_off_diff (Input), lp4x_ocd_40p_40n (I/O), lp4x_ocd_120p_120n (I/O), lp4x_ocd_48p_48n (I/O), lp4x_ocd_34p_34n (I/O), lp4x_ocd_80p_80n (I/O), lp4x_ocd_240p_240n (I/O), lp4x_ocd_60p_60n (I/O), lp4x_0p6_ocd_80p_80n (I/O)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
